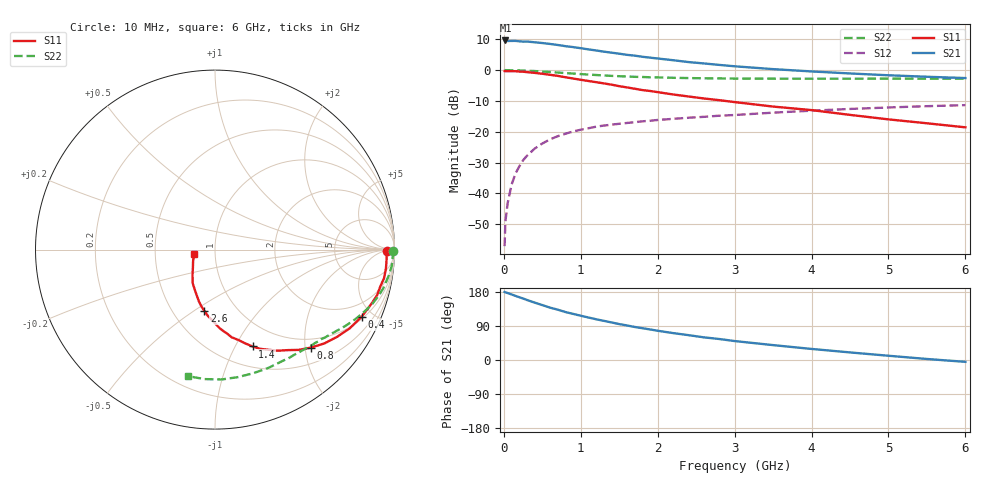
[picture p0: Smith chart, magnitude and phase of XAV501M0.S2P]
! SIEMENS Discrete & RF Semiconductors
! BFY180
! Si NPN RF Bipolar Junction Transistor in MICRO-X
! VCE = 0.5 V  IC = 1 mA
! Common Emitter S-Parameters:  May  1997
# GHz  S  MA  R  50
!  f  S11  S21  S12  S22
! GHz  MAG  ANG  MAG  ANG  MAG  ANG  MAG  ANG
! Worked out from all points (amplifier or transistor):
!   36 points, 10 MHz to 6 GHz, reference 50 ohm
!   highest |S21| = 9.6 dB at 20 MHz (marker M1)
!   |S21| within 3 dB of that: start of sweep to 1.131 GHz
!   unconditionally stable (mu >= 1): 2.067 GHz to end of sweep
!   at 250 MHz: K = 0.15, MSG = 19.2 dB, |S12| = -29.2 dB
!   at 1.4 GHz: K = 0.78, MSG = 11.7 dB, |S12| = -17.7 dB
!   at 6 GHz: K = 1.29, MAG = 1.1 dB, |S12| = -11.4 dB
!   S11 on the Smith chart (normalised r, x): 10 MHz: 47, -12; 400 MHz: 1.11, -4.31; 800 MHz: 0.81, -2.12; 1.4 GHz: 0.73, -1.18; 2.6 GHz: 0.71, -0.55; 6 GHz: 0.79, -0.04
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0.01  0.9606 -0.6  2.956 179.5  0.0014 84.9  0.9931 -0.3
0.02  0.9557 -1.2  3.009 178.5  0.0035 91.3  0.9947 -0.7
0.05  0.9576 -3.2  2.949 176.7  0.007 84.7  0.992 -1.7
0.1  0.9582 -6.2  2.958 173.0  0.0138 86.7  0.9899 -3.4
0.15  0.9552 -9.6  2.962 169.3  0.0208 83.4  0.9891 -5.1
0.25  0.9384 -15.7  2.882 162.3  0.0345 78.9  0.979 -8.5
0.3  0.9239 -18.8  2.891 158.4  0.0407 76.6  0.9723 -10.1
0.4  0.8985 -24.6  2.809 151.5  0.0532 72.6  0.961 -13.2
0.6  0.8363 -35.5  2.643 138.2  0.0752 64.5  0.9274 -19.0
0.8  0.7633 -45.7  2.433 126.6  0.0927 58.0  0.8907 -23.9
0.9  0.7274 -50.2  2.35 121.7  0.101 55.3  0.8753 -26.0
1.1  0.6634 -58.1  2.157 112.1  0.1138 50.4  0.8435 -30.1
1.4  0.5786 -68.8  1.909 99.1  0.1302 44.4  0.8029 -35.5
1.7  0.4975 -79.2  1.709 87.2  0.1426 40.2  0.775 -40.0
2  0.4379 -86.7  1.535 77.2  0.1551 36.7  0.7583 -44.6
2.2  0.4014 -91.2  1.44 71.0  0.1617 34.4  0.7475 -47.5
2.6  0.3458 -100.0  1.277 59.8  0.1742 30.9  0.7337 -53.0
3  0.3021 -107.3  1.148 50.0  0.1866 27.4  0.7257 -58.6
3.5  0.2555 -115.6  1.033 39.3  0.2036 23.8  0.7232 -65.5
4.5  0.1874 -132.0  0.879 20.0  0.2339 14.9  0.7218 -79.7
5.5  0.137 -153.0  0.777 2.7  0.2593 5.8  0.7238 -94.6
6  0.1178 -169.1  0.74 -4.9  0.2697 1.2  0.7209 -101.9
